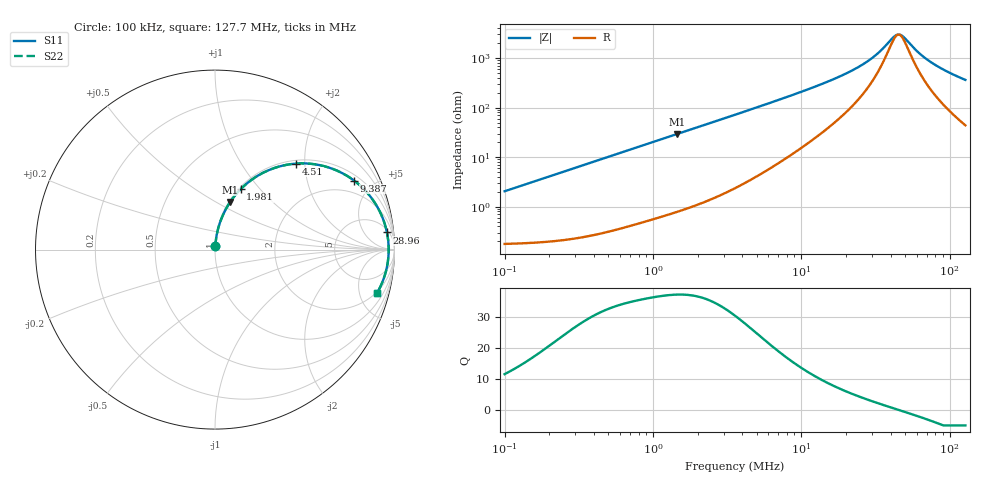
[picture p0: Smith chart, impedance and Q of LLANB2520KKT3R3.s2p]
! LLANB2520KKT3R3  S-PARAMETER MODEL  ( General Type )
! Model Generated by TAIYO YUDEN Corporation (http://www.ty-top.com)
! Version 1.0
! TAIYO YUDEN Control No. 160923NI42SB-FEC
! Copyright(c) 2016 TAIYO YUDEN CO.,LTD. All Rights Reserved.
! Product Description (link to TY-COMPAS)
! https://ds.yuden.co.jp/TYCOMPAS/or/detail?pn=LLANB2520KKT3R3M&u=M
! Products Name : Inductors
! Characteristics :
!  Inductance : 3.3 uH , SRF(min) : -Hz , DC Resistance(max) : 0.2 Ohm
!  Rated Current : Saturation :1550 mA , Temp Rise : 1300 mA (40 degC)
!  Case Size : 2.5 x 2.0 / 0.098 x 0.079 [mm/inch] , Thickness : 1 / 0.039 [mm/inch]
!  (Conditions: Temperature = 25 degC , DC Bias Current/Voltage = 0A / 0V)
! External Node Assignments :
!  1  o---GGG---o  2
! GND o---------o GND
! Frequency Range : 0.1MHz  -  127.746476MHz  [ 402 STEP ]
# MHz S RI R 50
! Freq[MHz].  S11 Real  S11 Imag  S21 Real  S21 Imag  S12 Real  S12 Imag  S22 Real  S22 Imag
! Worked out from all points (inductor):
!   401 points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, 100 kHz to 127.7 MHz, reference 50 ohm
!   read as one part in series: L = 3.25 uH near 103.6 kHz
!   highest Q = 37.2 at 1.462 MHz (marker M1), where L = 3.19 uH
!   self-resonance near 45.3 MHz
!   S11 on the Smith chart (normalised r, x): 100 kHz: 1.00, +0.04; 1.981 MHz: 1.02, +0.79; 4.51 MHz: 1.07, +1.81; 9.387 MHz: 1.27, +3.88; 28.96 MHz: 7, +18; 127.7 MHz: 1.88, -7.19
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0.1  0.00218 0.0203  0.9978 -0.0203  0.9978 -0.0203  0.00218 0.0203
0.33137  0.00688 0.0668  0.9931 -0.0668  0.9931 -0.0668  0.00688 0.0668
0.63079  0.0196 0.1247  0.9804 -0.1247  0.9804 -0.1247  0.0196 0.1247
1.098062  0.0517 0.2081  0.9483 -0.2081  0.9483 -0.2081  0.0517 0.2081
1.461776  0.0852 0.266  0.9148 -0.266  0.9148 -0.266  0.0852 0.266
1.981074  0.1426 0.3363  0.8574 -0.3363  0.8574 -0.3363  0.1426 0.3363
3.574164  0.344 0.4589  0.656 -0.4589  0.656 -0.4589  0.344 0.4589
4.509525  0.4528 0.4793  0.5472 -0.4793  0.5472 -0.4793  0.4528 0.4793
6.334063  0.617 0.4624  0.383 -0.4624  0.383 -0.4624  0.617 0.4624
9.387103  0.7756 0.384  0.2244 -0.384  0.2244 -0.384  0.7756 0.384
11.84371  0.8432 0.3224  0.1568 -0.3224  0.1568 -0.3224  0.8432 0.3224
19.8929  0.931 0.1839  0.069 -0.1839  0.069 -0.1839  0.931 0.1839
28.95886  0.9581 0.0953  0.0419 -0.0953  0.0419 -0.0953  0.9581 0.0953
34.01531  0.9639 0.0602  0.0361 -0.0602  0.0361 -0.0602  0.9639 0.0602
39.24654  0.9668 0.0299  0.0332 -0.0299  0.0332 -0.0299  0.9668 0.0299
43.69146  0.9676 0.00751  0.0324 -0.00751  0.0324 -0.00751  0.9676 0.00751
46.93103  0.9677 -0.00738  0.0323 0.00738  0.0323 0.00738  0.9677 -0.00738
49.51738  0.9674 -0.0186  0.0326 0.0186  0.0326 0.0186  0.9674 -0.0186
61.36888  0.9635 -0.0639  0.0365 0.0639  0.0365 0.0639  0.9635 -0.0639
73.38493  0.9566 -0.1032  0.0434 0.1032  0.0434 0.1032  0.9566 -0.1032
95.96105  0.9383 -0.1662  0.0617 0.1662  0.0617 0.1662  0.9383 -0.1662
127.7465  0.9041 -0.2398  0.0959 0.2398  0.0959 0.2398  0.9041 -0.2398
